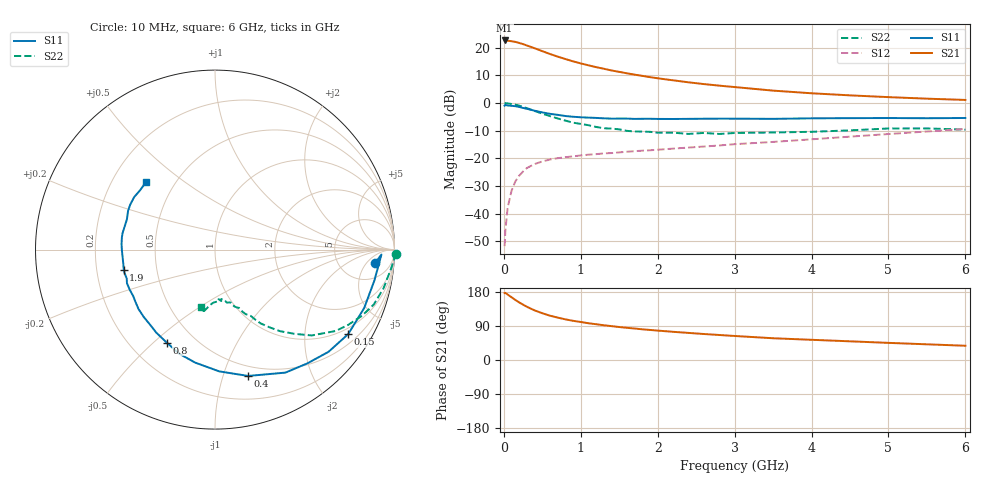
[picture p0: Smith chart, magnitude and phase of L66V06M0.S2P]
!  INFINEON TECHNOLOGIES Small Signal Semiconductors
! BFR380L3 , Si-NPN RF-Transistor in TSLP-3-1
!  Vce=6 V,  Ic=6 mA
! Common Emitter S-Parameters:  07. March 2005
#  GHz  S  MA  R  50
! f  S11  S21  S12  S22
! GHz  Mag  Ang  Mag  Ang  Mag  Ang  Mag  Ang
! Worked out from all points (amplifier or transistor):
!   36 points, 10 MHz to 6 GHz, reference 50 ohm
!   highest |S21| = 22.6 dB at 10 MHz (marker M1)
!   |S21| within 3 dB of that: start of sweep to 417.3 MHz
!   unconditionally stable (mu >= 1): 3.044 GHz to 4.542 GHz
!   at 250 MHz: K = 0.16, MSG = 23.0 dB, |S12| = -24.7 dB
!   at 1.4 GHz: K = 0.72, MSG = 14.9 dB, |S12| = -18.1 dB
!   at 6 GHz: K = 0.93, MSG = 5.2 dB, |S12| = -9.3 dB
!   S11 on the Smith chart (normalised r, x): 10 MHz: 12, -9; 150 MHz: 0.79, -3.27; 400 MHz: 0.41, -1.21; 800 MHz: 0.35, -0.55; 1.9 GHz: 0.32, -0.10; 6 GHz: 0.35, +0.37
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0.01  0.897 -4.6  13.54 176.6  0.0026 72.7  1.01 -1.3
0.02  0.9278 -1.7  13.42 177.2  0.005 91.3  1.001 -2.8
0.05  0.9045 -11.0  13.39 172.6  0.013 85.2  0.9853 -6.5
0.1  0.8927 -21.4  13.11 165.6  0.026 78.4  0.9635 -12.9
0.15  0.8789 -32.4  12.75 158.4  0.0385 72.7  0.9359 -19.1
0.2  0.8511 -42.0  12.21 151.9  0.0489 69.4  0.8985 -24.2
0.25  0.8165 -50.9  11.61 146.1  0.0581 64.1  0.8522 -29.5
0.3  0.7898 -60.2  10.98 140.4  0.0672 60.6  0.8109 -34.0
0.4  0.7278 -75.3  9.786 130.9  0.0792 54.7  0.7205 -41.6
0.5  0.6789 -88.0  8.674 123.4  0.0882 50.6  0.6446 -46.7
0.6  0.6394 -99.9  7.706 116.9  0.0957 47.6  0.5817 -51.4
0.8  0.5838 -117.4  6.252 107.3  0.1053 44.1  0.4827 -58.3
0.9  0.5665 -125.3  5.677 103.4  0.1091 43.4  0.4426 -60.5
1.1  0.5463 -136.6  4.81 97.0  0.1169 43.1  0.3982 -64.6
1.5  0.5251 -154.8  3.665 87.0  0.1286 44.2  0.3353 -71.1
1.9  0.521 -167.6  2.943 79.3  0.1404 46.4  0.3025 -77.4
2.2  0.5164 -175.0  2.579 74.4  0.1505 48.4  0.2923 -78.9
2.8  0.5233 172.4  2.067 66.0  0.1715 52.1  0.2767 -85.9
3.5  0.5189 161.1  1.68 57.4  0.1988 54.6  0.2942 -91.2
4.5  0.5346 152.2  1.379 49.3  0.2476 58.6  0.3218 -96.8
5.5  0.5327 141.8  1.202 41.4  0.3068 59.1  0.349 -101.8
6  0.538 135.5  1.14 37.6  0.341 58.3  0.3312 -103.9
